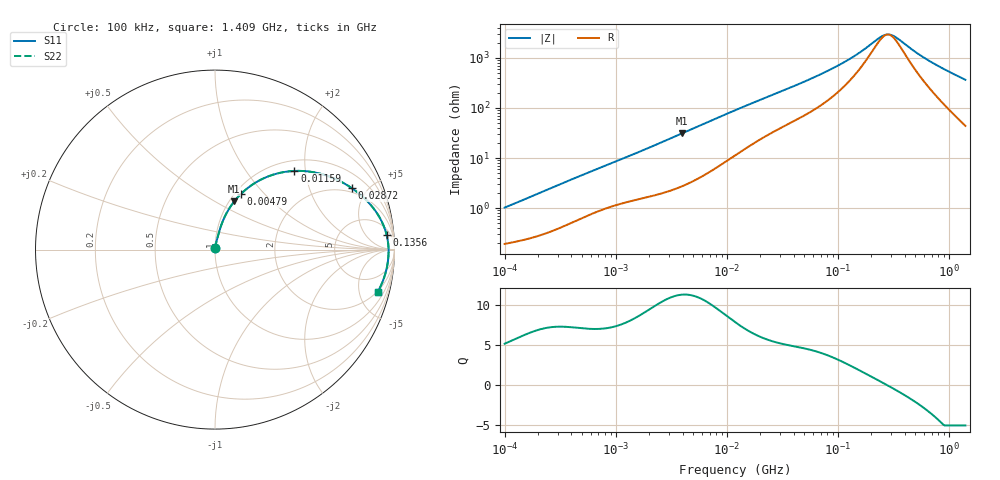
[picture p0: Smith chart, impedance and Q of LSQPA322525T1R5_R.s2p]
! LSQPA322525T1R5_R  S-PARAMETER MODEL  ( General Type )
! Model Generated by TAIYO YUDEN Corporation (http://www.ty-top.com)
! Version 2.0
! TAIYO YUDEN Control No. 100810NF25SB-HKC
! Copyright(c) 2007 TAIYO YUDEN CO.,LTD. All Rights Reserved.
! Product Description (link to TY-COMPAS)
! https://ds.yuden.co.jp/TYCOMPAS/or/detail?pn=LSQPA322525T1R5MR&u=M
! Products Name : Inductors
! Characteristics :
!  Inductance : 1.5 uH , SRF(min) : 220 MHz , DC Resistance(max) : 0.078 Ohm
!  Rated Current : Saturation :2000 mA , Temp Rise : 1310 mA (40 degC)
!  Case Size : 3.2 x 2.5 / 0.126 x 0.098 [mm/inch] , Thickness : 2.5 / 0.098 [mm/inch]
!  (Conditions: Temperature = 25 degC , DC Bias Current/Voltage = 0A / 0V)
! External Node Assignments :
!  1  o---GGG---o  2
! GND o---------o GND
! Frequency Range : 0.1MHz  -  1408.934139MHz  [ 402 STEP ]
# MHz S RI R 50
! Freq[MHz].  S11 Real  S11 Imag  S21 Real  S21 Imag  S12 Real  S12 Imag  S22 Real  S22 Imag
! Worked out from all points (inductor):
!   401 points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, 100 kHz to 1.409 GHz, reference 50 ohm
!   read as one part in series: L = 1.57 uH near 104.9 kHz
!   highest Q = 11.4 at 3.957 MHz (marker M1), where L = 1.25 uH
!   self-resonance near 281.6 MHz
!   S11 on the Smith chart (normalised r, x): 100 kHz: 1.00, +0.02; 4.79 MHz: 1.07, +0.75; 11.59 MHz: 1.22, +1.74; 28.72 MHz: 1.74, +3.95; 135.6 MHz: 9, +19; 1.409 GHz: 1.88, -7.25
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0.1  0.00202 0.01  0.998 -0.01  0.998 -0.01  0.00202 0.01
0.495381  0.00823 0.0443  0.9918 -0.0443  0.9918 -0.0443  0.00823 0.0443
1.227676  0.0226 0.0981  0.9774 -0.0981  0.9774 -0.0981  0.0226 0.0981
2.454022  0.0532 0.181  0.9468 -0.181  0.9468 -0.181  0.0532 0.181
3.956607  0.1076 0.2689  0.8924 -0.2689  0.8924 -0.2689  0.1076 0.2689
4.789616  0.1436 0.3092  0.8564 -0.3092  0.8564 -0.3092  0.1436 0.3092
7.18834  0.2563 0.3901  0.7437 -0.3901  0.7437 -0.3901  0.2563 0.3901
11.58972  0.4423 0.4382  0.5577 -0.4382  0.5577 -0.4382  0.4423 0.4382
12.15675  0.4622 0.4387  0.5378 -0.4387  0.5378 -0.4387  0.4622 0.4387
17.39406  0.605 0.4178  0.395 -0.4178  0.395 -0.4178  0.605 0.4178
28.7222  0.7629 0.3419  0.2371 -0.3419  0.2371 -0.3419  0.7629 0.3419
58.80098  0.8973 0.2104  0.1027 -0.2104  0.1027 -0.2104  0.8973 0.2104
92.56714  0.9386 0.1353  0.0614 -0.1353  0.0614 -0.1353  0.9386 0.1353
135.6477  0.9562 0.0823  0.0438 -0.0823  0.0438 -0.0823  0.9562 0.0823
240.6279  0.9663 0.0166  0.0337 -0.0166  0.0337 -0.0166  0.9663 0.0166
264.7493  0.9668 0.00651  0.0332 -0.00651  0.0332 -0.00651  0.9668 0.00651
291.2888  0.9671 -0.00358  0.0329 0.00358  0.0329 0.00358  0.9671 -0.00358
336.1686  0.967 -0.0188  0.033 0.0188  0.033 0.0188  0.967 -0.0188
504.5276  0.9635 -0.0651  0.0365 0.0651  0.0365 0.0651  0.9635 -0.0651
688.2146  0.9562 -0.1066  0.0438 0.1066  0.0438 0.1066  0.9562 -0.1066
1008.508  0.9374 -0.1696  0.0626 0.1696  0.0626 0.1696  0.9374 -0.1696
1408.934  0.9054 -0.2384  0.0946 0.2384  0.0946 0.2384  0.9054 -0.2384
